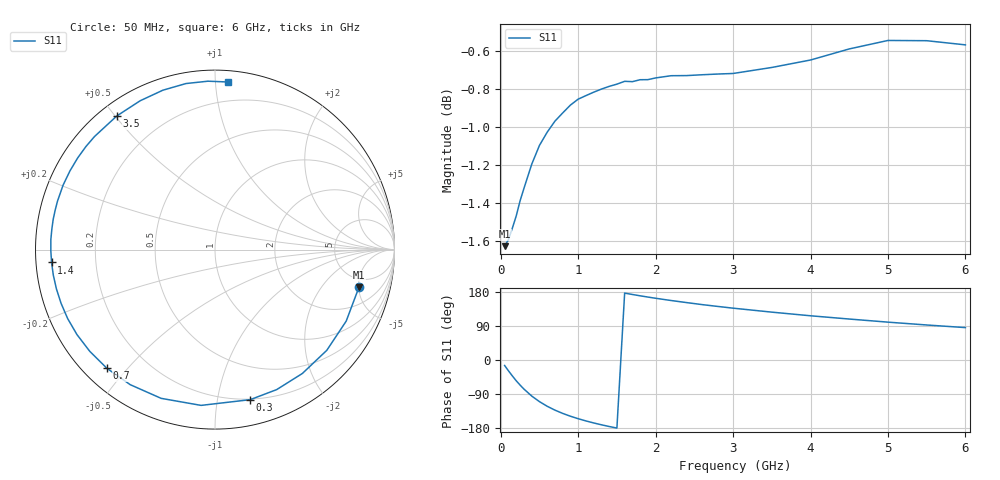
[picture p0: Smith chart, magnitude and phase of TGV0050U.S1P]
! SIEMENS Discrete & RF Semiconductors
! BAT64
! Si Schottky Diode in SOT23
! IF = 0.05 mA
! S-Parameters:  February  1997
# GHz  S  MA  R  50
!  f  S11
! GHz  MAG  ANG
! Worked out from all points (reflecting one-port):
!   34 points, 50 MHz to 6 GHz, reference 50 ohm
!   lowest |S11| = -1.6 dB at 50 MHz (marker M1), VSWR 10.71, Z = 190 - j253 ohm
!   phase of S11 starts at -15 deg and turns -260 deg over the sweep
!   S11 on the Smith chart (normalised r, x): 50 MHz: 3.81, -5.06; 300 MHz: 0.20, -1.24; 700 MHz: 0.07, -0.44; 1.4 GHz: 0.05, -0.04; 3.5 GHz: 0.05, +0.51; 6 GHz: 0.07, +1.08
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0.05  0.8292 -14.5
0.1  0.8326 -28.6
0.15  0.8383 -42.0
0.2  0.8446 -54.8
0.25  0.8523 -66.2
0.3  0.8588 -76.8
0.4  0.8714 -95.1
0.5  0.8814 -109.9
0.6  0.8885 -122.1
0.7  0.8944 -132.3
0.8  0.8989 -140.9
0.9  0.9032 -148.4
1  0.9064 -154.9
1.1  0.9084 -160.8
1.2  0.9102 -166.1
1.4  0.9134 -175.5
1.6  0.9163 176.5
1.8  0.9171 169.4
2  0.9181 162.9
2.4  0.9194 151.5
2.6  0.9199 146.2
3  0.9206 136.8
3.5  0.924 126.3
4  0.9282 116.7
4.5  0.9344 108.1
5  0.9392 99.9
5.5  0.9391 92.4
6  0.9367 85.5
